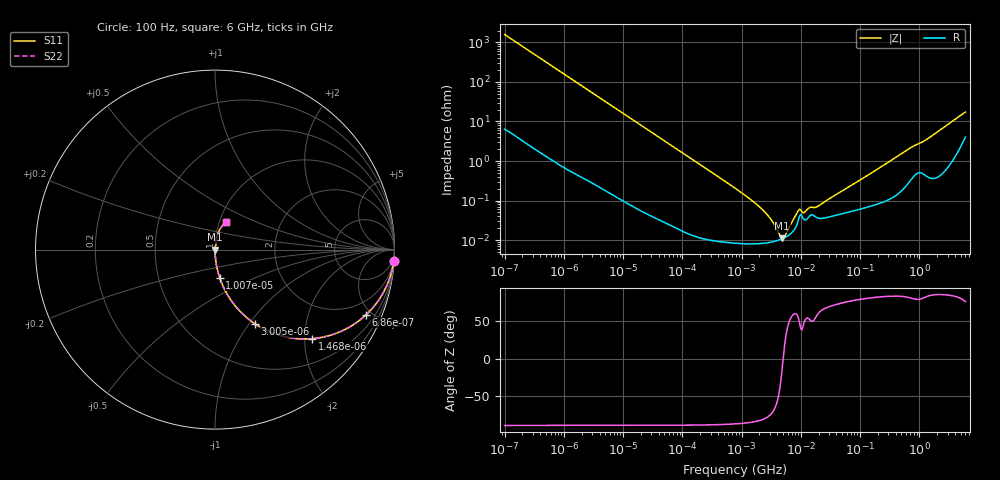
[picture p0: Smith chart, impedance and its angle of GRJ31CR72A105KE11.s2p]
!Murata Part Number: GRJ31CR72A105KE11
!These Parameters are Measured in Series Mode Connection
!Data Generated on Jun 19, 2026
!  o--ll--o
!Port1  Port2
!  o------o
!Operation Temp=25[degC], DC Bias Voltage=0[V]
!Freq. Start=100[Hz] Stop=6[GHz] 401[Steps]
# Hz S RI R 50
!Freq.(Hz) S11(Real) S11(Imag) S21(Real) S21(Imag) S12(Real) S12(Imag) S22(Real) S22(Imag)
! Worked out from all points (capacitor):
!   401 points, 100 Hz to 6 GHz, reference 50 ohm
!   read as one part in series: C = 1 uF near 109 Hz
!   lowest |Z| = 11.1 mohm at 4.857 MHz (marker M1)
!   series resonance near 5.039 MHz, so ESL is about 1 nH
!   S11 on the Smith chart (normalised r, x): 100 Hz: 1, -32; 686 Hz: 1.02, -4.65; 1.468 kHz: 1.01, -2.18; 3.005 kHz: 1.01, -1.07; 10.07 kHz: 1.00, -0.32; 6 GHz: 1.08, +0.34
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100  0.9958 -0.0627  0.0042 0.0627  0.0042 0.0627  0.9958 -0.0627
335  0.9569 -0.2011  0.0431 0.2011  0.0431 0.2011  0.9569 -0.2011
686  0.843 -0.3617  0.157 0.3617  0.157 0.3617  0.843 -0.3617
1468  0.5422 -0.496  0.4578 0.496  0.4578 0.496  0.5422 -0.496
2008  0.3887 -0.485  0.6113 0.485  0.6113 0.485  0.3887 -0.485
3005  0.2225 -0.4133  0.7775 0.4133  0.7775 0.4133  0.2225 -0.4133
5143  0.09 -0.2835  0.91 0.2835  0.91 0.2835  0.09 -0.2835
10066  0.0258 -0.1555  0.9742 0.1555  0.9742 0.1555  0.0258 -0.1555
40335  0.00193 -0.04  0.9981 0.04  0.9981 0.04  0.00193 -0.04
774597  8.75e-05 -0.00206  0.9999 0.00206  0.9999 0.00206  8.75e-05 -0.00206
2372521  8.34e-05 -0.000538  0.9999 0.000538  0.9999 0.000538  8.34e-05 -0.000538
3245845  8.96e-05 -0.000297  0.9999 0.000297  0.9999 0.000297  8.96e-05 -0.000297
4440638  0.000102 -8.33e-05  0.9999 8.33e-05  0.9999 8.33e-05  0.000102 -8.33e-05
4856642  0.000108 -2.43e-05  0.9999 2.43e-05  0.9999 2.43e-05  0.000108 -2.43e-05
5554849  0.000119 6.52e-05  0.9999 -6.52e-05  0.9999 -6.52e-05  0.000119 6.52e-05
9090158  0.000318 0.000457  0.9997 -0.000457  0.9997 -0.000457  0.000318 0.000457
1.137099e7  0.000328 0.000371  0.9997 -0.000371  0.9997 -0.000371  0.000328 0.000371
1.555665e7  0.000435 0.000518  0.9996 -0.000518  0.9996 -0.000518  0.000435 0.000518
1.946e7  0.00036 0.000622  0.9996 -0.000622  0.9996 -0.000622  0.00036 0.000622
3.124326e8  0.00116 0.00965  0.9988 -0.00965  0.9988 -0.00965  0.00116 0.00965
1.637704e9  0.00546 0.043  0.9945 -0.043  0.9945 -0.043  0.00546 0.043
6e9  0.0631 0.1512  0.9369 -0.1512  0.9369 -0.1512  0.0631 0.1512
